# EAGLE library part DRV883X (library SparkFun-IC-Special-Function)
DRV8835 2 Channel Motor Driver Dual 1.5A H-bridge, 2-11V Datasheet SparkFun Products: SparkFun Serial Controlled Motor Driver
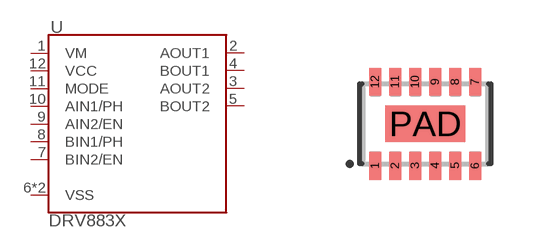
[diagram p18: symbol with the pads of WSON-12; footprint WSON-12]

Designator prefix U

## DRV883X (PROD_ID: IC-13342; VALUE: DRV8835)  [WSON-12]
1  VM
2  AOUT1
3  AOUT2
4  BOUT1
5  BOUT2
6  VSS
7  BIN2/EN
8  BIN1/PH
9  AIN2/EN
10  AIN1/PH
11  MODE
12  VCC
PAD  VSS

## Footprint WSON-12 (pad centres in mm)
WSON-12 Specifications: Pin count: 12 Area:2mmx3mm Datasheet referenced for footprint Example device(s): DRV883X
smd 0.3 x 0.7: 1 -1.25,-1.05; 2 -0.75,-1.05; 3 -0.25,-1.05; 4 0.25,-1.05; 5 0.75,-1.05; 6 1.25,-1.05; 7 1.25,1.05; 8 0.75,1.05; 9 0.25,1.05; 10 -0.25,1.05; 11 -0.75,1.05; 12 -1.25,1.05
smd 2 x 0.9: PAD 0,0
